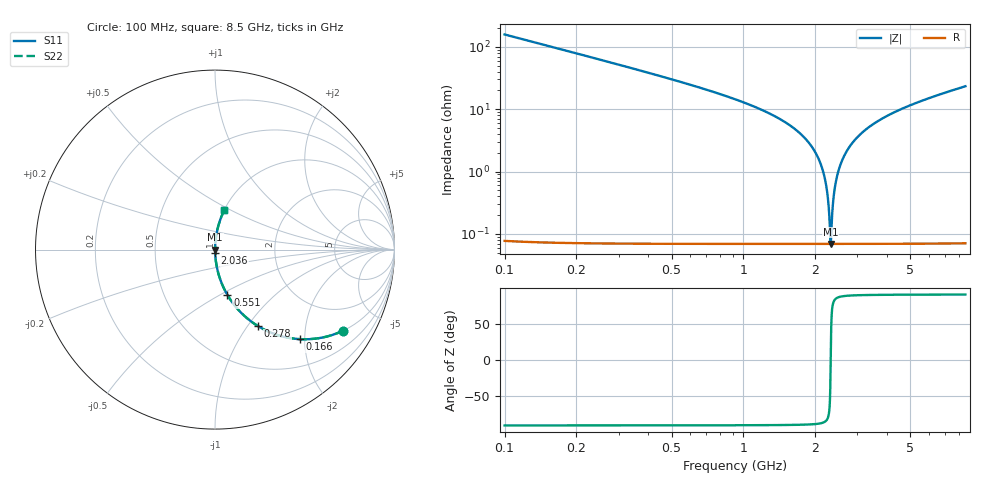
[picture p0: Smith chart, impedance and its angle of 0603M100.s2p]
! Created Wed Apr 18 16:35:35 2012
# hz S ma R 50
! 2 Port Network Data from SP1.SP block
! freq  magS11  angS11  magS21  angS21  magS12  angS12  magS22  angS22
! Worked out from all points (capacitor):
!   8401 points, 100 MHz to 8.5 GHz, reference 50 ohm
!   read as one part in series: C = 10 pF near 142 MHz
!   lowest |Z| = 69.1 mohm at 2.319 GHz (marker M1)
!   series resonance near 2.319 GHz, so ESL is about 470 pH
!   S11 on the Smith chart (normalised r, x): 100 MHz: 1.00, -3.16; 166 MHz: 1.00, -1.90; 278 MHz: 1.00, -1.12; 551 MHz: 1.00, -0.54; 2.036 GHz: 1.00, -0.04; 8.5 GHz: 1.00, +0.47
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1e8  0.8449 -32.3  0.5345 57.7  0.5345 57.7  0.8449 -32.3
1.66e8  0.6882 -46.5  0.725 43.5  0.725 43.5  0.6882 -46.5
2.78e8  0.4893 -60.6  0.8715 29.3  0.8715 29.3  0.4893 -60.6
5.51e8  0.2616 -74.7  0.9645 15.2  0.9645 15.2  0.2616 -74.7
1.5e9  0.06128 -85.8  0.9974 3.5  0.9974 3.5  0.06128 -85.8
1.819e9  0.03349 -86.9  0.9988 1.9  0.9988 1.9  0.03349 -86.9
2.036e9  0.01785 -86.8  0.9992 1.0  0.9992 1.0  0.01785 -86.8
2.202e9  0.00713 -84.0  0.9993 0.4  0.9993 0.4  0.00713 -84.0
2.249e9  0.004267 -80.5  0.9993 0.2  0.9993 0.2  0.004267 -80.5
2.295e9  0.001602 -64.4  0.9993 0.1  0.9993 0.1  0.001602 -64.4
2.319e9  0.00069 -2.1  0.9993 0.0  0.9993 0.0  0.00069 -2.1
2.345e9  0.001648 65.2  0.9993 -0.1  0.9993 -0.1  0.001648 65.2
2.383e9  0.003756 79.2  0.9993 -0.2  0.9993 -0.2  0.003756 79.2
2.413e9  0.005445 82.4  0.9993 -0.3  0.9993 -0.3  0.005445 82.4
2.502e9  0.01038 85.6  0.9993 -0.6  0.9993 -0.6  0.01038 85.6
2.663e9  0.01893 86.8  0.9991 -1.1  0.9991 -1.1  0.01893 86.8
2.9e9  0.03076 87.0  0.9988 -1.8  0.9988 -1.8  0.03076 87.0
3.454e9  0.05578 86.1  0.9978 -3.2  0.9978 -3.2  0.05578 86.1
4.3e9  0.08951 84.4  0.9953 -5.1  0.9953 -5.1  0.08951 84.4
5.7e9  0.1391 81.7  0.9896 -8.0  0.9896 -8.0  0.1391 81.7
7.1e9  0.1844 79.2  0.9822 -10.6  0.9822 -10.6  0.1844 79.2
8.5e9  0.2273 76.7  0.9731 -13.1  0.9731 -13.1  0.2273 76.7
